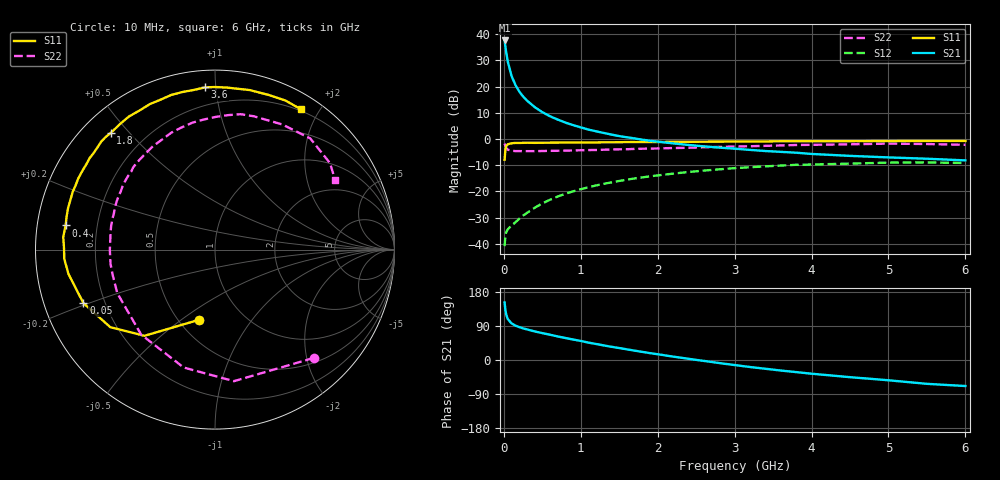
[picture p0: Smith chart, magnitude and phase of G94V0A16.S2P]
! SIEMENS Small Signal Semiconductors
! BFG235
! Si NPN RF Bipolar Junction Transistor in SOT223
! VCE = 4 V  IC = 160 mA
! Common Emitter S-Parameters:  July  1994
# GHz  S  MA  R  50
!  f  S11  S21  S12  S22
! GHz  MAG  ANG  MAG  ANG  MAG  ANG  MAG  ANG
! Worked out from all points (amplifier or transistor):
!   40 points, 10 MHz to 6 GHz, reference 50 ohm
!   highest |S21| = 37.6 dB at 10 MHz (marker M1)
!   |S21| within 3 dB of that: start of sweep to 23.81 MHz
!   unconditionally stable (mu >= 1): 433.7 MHz to 1.521 GHz
!   at 200 MHz: K = 0.82, MSG = 24.3 dB, |S12| = -30.5 dB
!   at 1.5 GHz: K = 1.00, MAG = 8.2 dB, |S12| = -16.0 dB
!   at 6 GHz: K = 0.90, MSG = 0.5 dB, |S12| = -9.2 dB
!   S11 on the Smith chart (normalised r, x): 10 MHz: 0.62, -0.58; 50 MHz: 0.12, -0.19; 400 MHz: 0.09, +0.08; 1.8 GHz: 0.08, +0.44; 3.6 GHz: 0.09, +0.94; 6 GHz: 0.18, +1.77
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0.01  0.4023 -103.1  75.94 151.7  0.009 61.2  0.8163 -47.7
0.02  0.6207 -129.3  59.15 132.4  0.0142 48.2  0.7406 -81.8
0.03  0.7262 -143.5  46.01 120.7  0.0166 40.9  0.6797 -104.9
0.05  0.7916 -157.9  30.45 108.4  0.0188 34.3  0.6273 -131.0
0.1  0.8277 -170.6  16.04 96.6  0.0223 37.6  0.596 -156.0
0.15  0.8417 -176.6  10.76 90.6  0.0256 44.3  0.5874 -166.4
0.2  0.8407 -179.6  8.051 86.9  0.03 48.8  0.5874 -172.2
0.25  0.8439 177.4  6.482 83.4  0.0345 52.6  0.5854 -176.3
0.3  0.8485 175.3  5.413 80.8  0.0388 54.6  0.5859 -179.8
0.4  0.8434 170.8  4.075 75.5  0.0486 57.5  0.5857 175.2
0.5  0.8471 167.3  3.254 70.9  0.0589 58.6  0.5894 171.0
0.7  0.8522 160.5  2.345 62.1  0.0797 57.8  0.5966 163.7
0.9  0.8552 155.2  1.839 54.0  0.1001 54.9  0.6039 157.5
1.1  0.8596 148.8  1.512 45.8  0.12 51.4  0.614 151.2
1.4  0.8642 141.6  1.213 34.8  0.1484 45.3  0.6295 142.8
1.8  0.8717 131.8  0.969 21.4  0.1849 36.6  0.6517 131.7
2.2  0.883 122.9  0.824 8.9  0.218 27.6  0.6719 121.0
3.2  0.8965 101.5  0.619 -18.5  0.2889 4.3  0.7272 95.1
3.6  0.9055 93.5  0.568 -27.8  0.3108 -5.5  0.7534 84.2
4.5  0.9095 77.8  0.476 -45.3  0.339 -25.2  0.7915 61.8
5.5  0.9186 64.7  0.42 -62.9  0.3569 -47.0  0.8017 36.9
6  0.9167 58.6  0.39 -68.7  0.3474 -55.0  0.773 30.0
